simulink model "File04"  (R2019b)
settings: Solver=FixedStepDiscrete  StartTime=0.0  StopTime=50  FixedStep=1  RelTol=1e-3

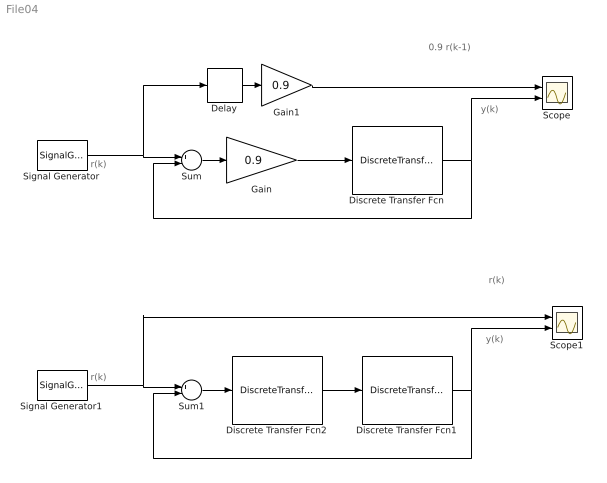
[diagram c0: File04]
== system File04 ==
  note: r(k)
  note: 0.9 r(k-1)
  note: r(k)
  note: r(k)
  note: y(k)
  note: y(k)
  Delay : Delay  DelayLength=1
  Discrete Transfer Fcn : DiscreteTransferFcn  Denominator=[1 -0.9]
  Discrete Transfer Fcn1 : DiscreteTransferFcn  Denominator=[1 -0.9]
  Discrete Transfer Fcn2 : DiscreteTransferFcn  Numerator=[1 -0.9]  Denominator=[1 -1]
  Gain : Gain  Gain=0.9
  Gain1 : Gain  Gain=0.9
  Scope : Scope  NumInputPorts=2
  Scope1 : Scope  NumInputPorts=2
  Signal Generator : SignalGenerator  Units=rad/sec
  Signal Generator1 : SignalGenerator  Units=rad/sec
  Sum : Sum  Inputs=+-
  Sum1 : Sum  Inputs=+-
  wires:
  Discrete Transfer Fcn/1 -> Scope/2, Sum/2
  Signal Generator/1 -> Delay/1, Sum/1
  Sum/1 -> Gain/1
  Gain/1 -> Discrete Transfer Fcn/1
  Delay/1 -> Gain1/1
  Gain1/1 -> Scope/1
  Signal Generator1/1 -> Scope1/1, Sum1/1
  Discrete Transfer Fcn2/1 -> Discrete Transfer Fcn1/1
  Sum1/1 -> Discrete Transfer Fcn2/1
  Discrete Transfer Fcn1/1 -> Sum1/2, Scope1/2
